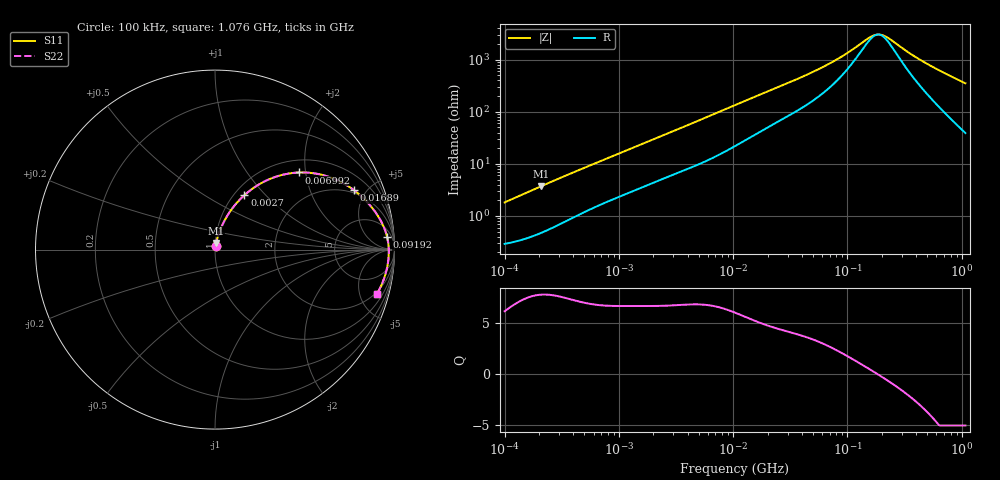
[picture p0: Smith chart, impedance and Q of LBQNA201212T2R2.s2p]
! LBQNA201212T2R2  S-PARAMETER MODEL  ( General Type )
! Model Generated by TAIYO YUDEN Corporation (http://www.ty-top.com)
! Version 1.0
! TAIYO YUDEN Control No. 191025NI43SB-FBB
! Copyright(c) 2019 TAIYO YUDEN CO.,LTD. All Rights Reserved.
! Product Description (link to TY-COMPAS)
! https://ds.yuden.co.jp/TYCOMPAS/or/detail?pn=LBQNA201212T2R2M&u=M
! Products Name : Inductors
! Characteristics :
!  Inductance : 2.2 uH , SRF(min) : 80 MHz , DC Resistance(max) : 0.299 Ohm
!  Rated Current : Saturation :410 mA , Temp Rise : 620 mA (20 degC)
!  Case Size : 2.0 x 1.25 / 0.079 x 0.049 [mm/inch] , Thickness : 1.25 / 0.049 [mm/inch]
!  (Conditions: Temperature = 25 degC , DC Bias Current/Voltage = 0A / 0V)
! External Node Assignments :
!  1  o---GGG---o  2
! GND o---------o GND
! Frequency Range : 0.1MHz  -  1076.144768MHz  [ 402 STEP ]
# MHz S RI R 50
! Freq[MHz].  S11 Real  S11 Imag  S21 Real  S21 Imag  S12 Real  S12 Imag  S22 Real  S22 Imag
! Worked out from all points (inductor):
!   401 points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, 100 kHz to 1.076 GHz, reference 50 ohm
!   read as one part in series: L = 2.85 uH near 104.8 kHz
!   highest Q = 7.82 at 210.2 kHz (marker M1), where L = 2.82 uH
!   self-resonance near 185.2 MHz
!   S11 on the Smith chart (normalised r, x): 100 kHz: 1.01, +0.04; 2.7 MHz: 1.11, +0.77; 6.992 MHz: 1.28, +1.84; 16.89 MHz: 1.81, +4.13; 91.92 MHz: 12, +21; 1.076 GHz: 1.78, -7.00
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0.1  0.00322 0.0179  0.9968 -0.0179  0.9968 -0.0179  0.00322 0.0179
0.21016  0.0061 0.0368  0.9939 -0.0368  0.9939 -0.0368  0.0061 0.0368
0.47352  0.0172 0.0773  0.9828 -0.0773  0.9828 -0.0773  0.0172 0.0773
1.1707  0.055 0.1653  0.945 -0.1653  0.945 -0.1653  0.055 0.1653
2.242212  0.1288 0.2687  0.8712 -0.2687  0.8712 -0.2687  0.1288 0.2687
2.699691  0.1634 0.3029  0.8366 -0.3029  0.8366 -0.3029  0.1634 0.3029
4.195927  0.2786 0.3813  0.7214 -0.3813  0.7214 -0.3813  0.2786 0.3813
6.991669  0.4688 0.4296  0.5312 -0.4296  0.5312 -0.4296  0.4688 0.4296
10.37374  0.6246 0.4086  0.3754 -0.4086  0.3754 -0.4086  0.6246 0.4086
16.88918  0.7745 0.331  0.2255 -0.331  0.2255 -0.331  0.7745 0.331
27.49678  0.8682 0.2417  0.1318 -0.2417  0.1318 -0.2417  0.8682 0.2417
49.12173  0.9301 0.1484  0.0699 -0.1484  0.0699 -0.1484  0.9301 0.1484
67.98125  0.9489 0.1045  0.0511 -0.1045  0.0511 -0.1045  0.9489 0.1045
91.92316  0.9593 0.0691  0.0407 -0.0691  0.0407 -0.0691  0.9593 0.0691
149.6574  0.9671 0.0199  0.0329 -0.0199  0.0329 -0.0199  0.9671 0.0199
172.0189  0.968 0.00687  0.032 -0.00687  0.032 -0.00687  0.968 0.00687
197.7217  0.9684 -0.00615  0.0316 0.00615  0.0316 0.00615  0.9684 -0.00615
232.6012  0.9683 -0.0215  0.0317 0.0215  0.0317 0.0215  0.9683 -0.0215
345.1171  0.9653 -0.062  0.0347 0.062  0.0347 0.062  0.9653 -0.062
466.6619  0.9593 -0.0987  0.0407 0.0987  0.0407 0.0987  0.9593 -0.0987
725.2975  0.9399 -0.1669  0.0601 0.1669  0.0601 0.1669  0.9399 -0.1669
1076.145  0.902 -0.2467  0.098 0.2467  0.098 0.2467  0.902 -0.2467
